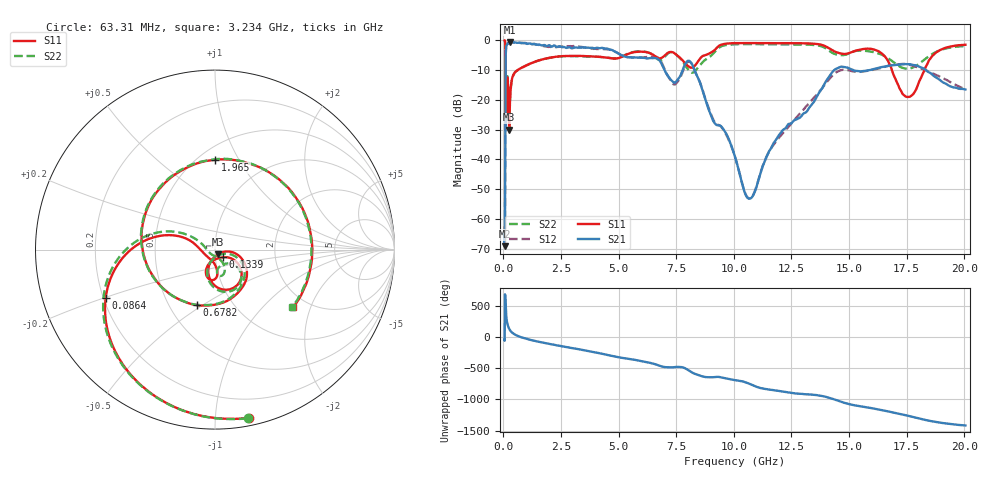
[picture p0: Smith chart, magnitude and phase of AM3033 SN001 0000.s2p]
# Hz S DB R 50
!freq MagS11 AngS11 MagS21 AngS21 MagS12 AngS12 MagS22 AngS22
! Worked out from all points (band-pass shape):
!   1601 points, 50 MHz to 20.05 GHz, reference 50 ohm
!   highest |S21| = -0.68 dB at 290.8 MHz (marker M1); lowest = -69.1 dB at 50.38 MHz (marker M2)
!   |S21| within 3 dB of the highest: 104.6 MHz to 4.786 GHz (4.682 GHz wide, 191 % of centre)
!   lowest |S11| = -30.1 dB at 248.5 MHz (marker M3), VSWR 1.06, Z = 51.5 - j2.81 ohm
!   |S11| at or under -10 dB: 91.78 MHz to 629 MHz (537.3 MHz wide, 149 % of centre); 16.86 GHz to 18.28 GHz (1.42 GHz wide, 8.08 % of centre)
!   |S22| runs from -29.7 to -0.1 dB; largest |S21 - S12| = 0.062
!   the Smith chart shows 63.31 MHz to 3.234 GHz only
!   S11 on the Smith chart (normalised r, x): 63.31 MHz: 0.06, -1.22; 86.4 MHz: 0.21, -0.20; 133.9 MHz: 1.09, -0.09; 678.2 MHz: 0.68, -0.47; 1.965 GHz: 0.60, +0.80; 3.234 GHz: 1.69, -1.53
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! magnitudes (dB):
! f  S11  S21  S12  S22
! 50 MHz  -0.2  -68.4  -62.5  -0.1
! 50.38 MHz  -0.2  -69.1  -63.7  -0.2
! 63.31 MHz  -0.4  -66.3  -66.0  -0.4
! 86.4 MHz  -3.5  -19.2  -19.2  -3.6
! 99.99 MHz  -23.8  -4.6  -4.6  -29.7
! 133.9 MHz  -24.2  -1.8  -1.8  -19.5
! 135.9 MHz  -22.3  -1.8  -1.8  -18.6
! 179.4 MHz  -12.9  -1.3  -1.3  -12.5
! 248.5 MHz  -30.1  -0.7  -0.7  -28.3
! 290.8 MHz  -19.1  -0.7  -0.7  -19.3
! 369.6 MHz  -13.1  -0.8  -0.7  -13.2
! 678.2 MHz  -9.7  -0.9  -0.9  -9.8
! 1.005 GHz  -8.5  -1.3  -1.1  -8.4
! 1.965 GHz  -6.0  -1.7  -2.3  -6.0
! 2.722 GHz  -5.3  -2.6  -2.2  -5.4
! 3.234 GHz  -5.3  -2.6  -2.2  -5.4
! 7.402 GHz  -4.3  -14.2  -14.9  -4.3
! 8.251 GHz  -9.0  -9.3  -9.4  -10.8
! 10.69 GHz  -1.0  -53.2  -53.1  -1.4
! 14.53 GHz  -4.3  -9.3  -10.5  -5.0
! 17.59 GHz  -19.1  -8.1  -8.2  -9.6
! 20.05 GHz  -1.6  -16.6  -16.4  -2.0
